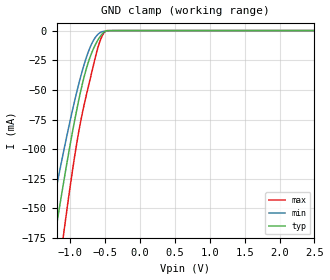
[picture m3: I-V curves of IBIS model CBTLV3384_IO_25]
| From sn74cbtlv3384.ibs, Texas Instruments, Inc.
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[Model]   CBTLV3384_IO_25
Model_type  Terminator
| variable   typ   min   max
C_comp   10pF   NA   NA
| C_tri-state   5.36pF   4.53pF   5.95pF
[Temperature Range]   40   100   -40
| Ambient temperature   25   85   -40
[Voltage range]   2.5   2.3   2.7
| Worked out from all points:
|   GND clamp passes 1 mA (typ) near -0.51 V on its own axis
[GND Clamp]
| CBTLV3384_IO_25
|   Voltage   I(typ)   I(min)   I(max)
-2.5V     -699.7mA   -574.4mA   -888.4mA
-1.325V   -211.3mA   -170.2mA   -276.9mA
-1.205V   -166.3mA   -133.2mA   -220.1mA
-1.105V   -130.3mA   -103.8mA   -174.6mA
-1.085V   -123.4mA   -98.1mA    -165.8mA
-930mV    -72.8mA    -56.75mA   -102.3mA
-815mV    -41.57mA   -30.79mA   -65.61mA
-695mV    -18.77mA   -11.11mA   -35.32mA
-575mV    -5.12mA    -1.718mA   -8.701mA
-520mV    -1.362mA   -622.9uA   -2.028mA
-475mV    -72.05uA   -328.9uA   -50.52uA
2.5V      1.258nA    61.07nA    12.54pA
